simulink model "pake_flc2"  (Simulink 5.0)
settings: Solver=ode45  StartTime=0.0  StopTime=1000  RelTol=1e-6
undefined symbols (not defined in the file or in its folder): fiskeretasug2
libraries: fuzwiz x1

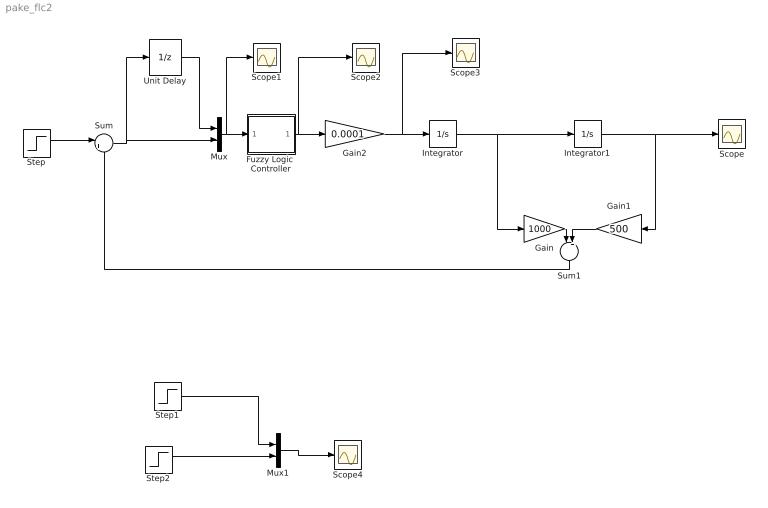
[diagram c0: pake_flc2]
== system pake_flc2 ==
  Fuzzy Logic  Controller : Subsystem  AncestorBlock="fuzblock/Fuzzy Logic  Controller"  mask(FIS){fis=fiskeretasug2}
      mask prompts: fis "FIS File or Structure:"
      mask help: FIS
      mask init:
      | fis = fuzblockmask(gcb,fis);
  Gain : Gain  Gain=1000
  Gain1 : Gain  Orientation=left  Gain=500
  Gain2 : Gain  Gain=0.0001
  Integrator : Integrator
  Integrator1 : Integrator
  Mux : Mux  Inputs=2
  Mux1 : Mux  Inputs=2
  Scope{,1..4} (5 alike) : Scope
  Step : Step  After=100  SampleTime=1
  Step1 : Step  After=10  SampleTime=1
  Step2 : Step  Before=5  After=20  SampleTime=1
  Sum : Sum  Inputs=|+-
  Sum1 : Sum  Orientation=down  Inputs=|++
  Unit Delay : UnitDelay
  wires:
  Gain1/1 -> Sum1/2
  Gain/1 -> Sum1/1
  Integrator/1 -> Gain/1, Integrator1/1
  Mux/1 -> Fuzzy Logic  Controller/1(In1), Scope1/1
  Fuzzy Logic  Controller/1(Out1) -> Gain2/1, Scope2/1
  Gain2/1 -> Integrator/1, Scope3/1
  Integrator1/1 -> Gain1/1, Scope/1
  Unit Delay/1 -> Mux/1
  Sum/1 -> Mux/2, Unit Delay/1
  Sum1/1 -> Sum/2
  Step/1 -> Sum/1
  Mux1/1 -> Scope4/1
  Step1/1 -> Mux1/1
  Step2/1 -> Mux1/2

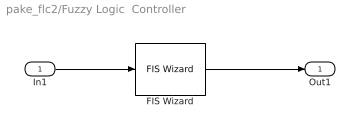
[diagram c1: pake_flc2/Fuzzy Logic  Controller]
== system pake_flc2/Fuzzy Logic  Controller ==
  In1 : Inport
  FIS Wizard : fuzwiz/FIS Wizard  fis=fis
  Out1 : Outport
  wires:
  In1/1 -> FIS Wizard/1
  FIS Wizard/1 -> Out1/1
